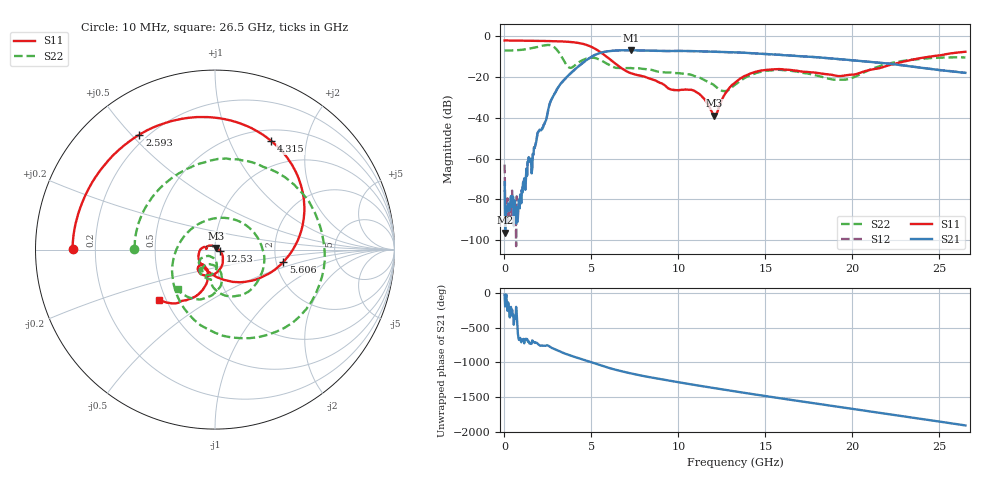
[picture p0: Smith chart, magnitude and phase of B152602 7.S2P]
!  2-Port S-parameters saved by WinCal
! VAR MeasName=S-Parameters (CALIBRATED_DATA) read from VNA (N5242A)
! VAR MeasDate=2016-1-5 16:26:33
! VAR NAME=B152602 7
! VAR FILENAME=B152602 7.S2P
! VAR DATE=2016-1-5 16:26:33
! VAR PHYS_PORTS=1,2
# Hz S DB R 50
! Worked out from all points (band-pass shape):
!   801 points, 10 MHz to 26.5 GHz, reference 50 ohm
!   highest |S21| = -6.77 dB at 7.262 GHz (marker M1); lowest = -96.3 dB at 43.11 MHz (marker M2)
!   |S21| within 3 dB of the highest: 5.055 GHz to 17.07 GHz (12.01 GHz wide, 109 % of centre)
!   lowest |S11| = -38.9 dB at 12.06 GHz (marker M3), VSWR 1.02, Z = 50.7 + j0.916 ohm
!   |S11| at or under -10 dB: 5.878 GHz to 24.4 GHz (18.52 GHz wide, 122 % of centre)
!   |S22| runs from -26.9 to -4.2 dB; largest |S21 - S12| = 0.0029
!   S11 on the Smith chart (normalised r, x): 10 MHz: 0.12, +0.00; 2.593 GHz: 0.17, +0.53; 4.315 GHz: 0.64, +1.44; 5.606 GHz: 2.18, -0.36; 12.53 GHz: 1.06, -0.01; 26.5 GHz: 0.46, -0.31
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1e7  -2.01 179.7  -71.53 -25.8  -62.89 -81.8  -6.96 179.4
4.31125e7  -2.01 179.1  -96.35 166.3  -80.86 -86.2  -6.97 177.4
1.755625e8  -2.02 176.4  -85.90 102.5  -79.42 123.8  -6.95 169.2
8.70925e8  -2.09 162.1  -84.42 55.6  -81.76 18.5  -6.70 126.0
1.8643e9  -2.22 141.0  -49.53 -1.0  -49.58 -0.8  -5.27 54.6
2.592775e9  -2.31 123.3  -33.31 -52.0  -33.32 -52.0  -4.25 -23.6
2.9239e9  -2.38 114.1  -27.63 -95.5  -27.65 -95.5  -5.77 -73.6
3.32125e9  -2.50 102.0  -22.37 -139.6  -22.38 -139.7  -10.48 -140.6
4.314625e9  -3.33 62.7  -14.27 134.8  -14.29 134.9  -12.48 23.2
4.447075e9  -3.55 56.2  -13.39 124.0  -13.40 124.1  -11.86 8.4
5.606012e9  -8.26 -10.5  -7.88 28.8  -7.88 28.9  -12.00 -81.5
7.261638e9  -18.03 -109.9  -6.77 -80.0  -6.77 -80.1  -15.54 -106.3
8.851038e9  -22.43 175.4  -7.08 -158.0  -7.07 -158.1  -17.36 -127.7
1.100335e10  -27.18 153.4  -7.27 110.2  -7.28 110.2  -19.66 -144.3
1.206295e10  -38.89 52.7  -7.56 67.7  -7.57 67.6  -24.04 -143.7
1.252652e10  -30.75 -12.5  -7.64 49.3  -7.62 49.2  -26.72 -124.8
1.3255e10  -22.67 -53.6  -7.85 20.6  -7.85 20.5  -23.74 -86.9
1.553976e10  -16.16 -114.4  -8.91 -67.1  -8.87 -67.3  -16.49 -107.1
1.769208e10  -17.64 -134.2  -10.08 -147.4  -10.06 -147.4  -18.69 -124.2
1.964571e10  -19.02 -118.9  -11.45 140.8  -11.42 140.6  -21.16 -94.2
2.209604e10  -14.17 -104.0  -13.42 51.1  -13.36 51.0  -13.28 -84.0
2.65e10  -7.56 -137.6  -17.90 -111.0  -17.90 -111.5  -10.34 -133.4
